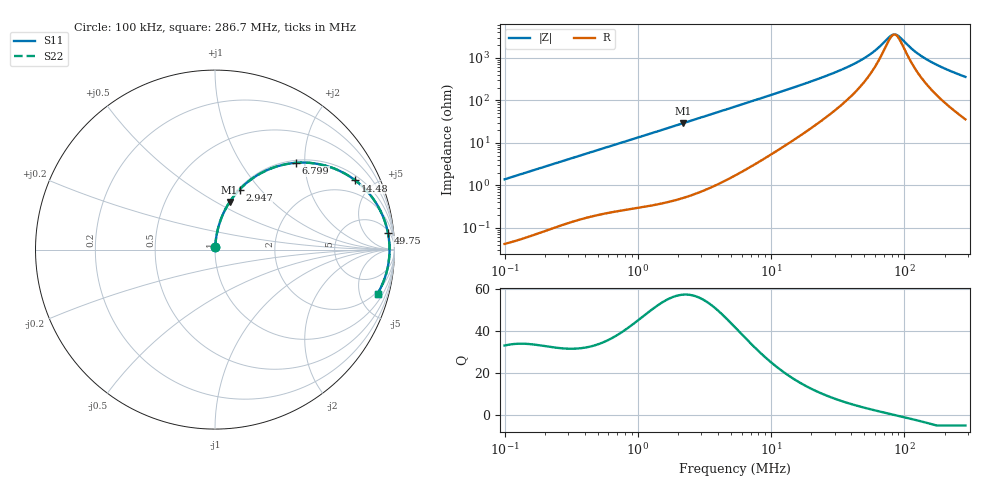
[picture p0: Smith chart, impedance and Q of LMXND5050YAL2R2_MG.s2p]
! LMXND5050YAL2R2_MG  S-PARAMETER MODEL  ( General Type )
! Model Generated by TAIYO YUDEN Corporation (http://www.ty-top.com)
! Version 1.0
! TAIYO YUDEN Control No. 191023NI43SB-FBB
! Copyright(c) 2019 TAIYO YUDEN CO.,LTD. All Rights Reserved.
! Product Description (link to TY-COMPAS)
! https://ds.yuden.co.jp/TYCOMPAS/or/detail?pn=LMXND5050YAL2R2NMG&u=M
! Products Name : Inductors
! Characteristics :
!  Inductance : 2.2 uH , SRF(min) : 42 MHz , DC Resistance(max) : 0.0286 Ohm
!  Rated Current : Saturation :5000 mA , Temp Rise : 3700 mA
!  Case Size : 4.9 x 4.9 / 0.193 x 0.193 [mm/inch] , Thickness : 4.1 / 0.161 [mm/inch]
!  (Conditions: Temperature = 25 degC , DC Bias Current/Voltage = 0A / 0V)
! External Node Assignments :
!  1  o---GGG---o  2
! GND o---------o GND
! Frequency Range : 0.1MHz  -  286.687601MHz  [ 402 STEP ]
# MHz S RI R 50
! Freq[MHz].  S11 Real  S11 Imag  S21 Real  S21 Imag  S12 Real  S12 Imag  S22 Real  S22 Imag
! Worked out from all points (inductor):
!   401 points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, 100 kHz to 286.7 MHz, reference 50 ohm
!   read as one part in series: L = 2.2 uH near 104.1 kHz
!   highest Q = 57.4 at 2.186 MHz (marker M1), where L = 2.11 uH
!   self-resonance near 84.18 MHz
!   S11 on the Smith chart (normalised r, x): 100 kHz: 1.00, +0.03; 2.947 MHz: 1.01, +0.78; 6.799 MHz: 1.05, +1.81; 14.48 MHz: 1.22, +3.93; 49.75 MHz: 6, +19; 286.7 MHz: 1.71, -7.08
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0.1  0.00061 0.0138  0.9994 -0.0138  0.9994 -0.0138  0.00061 0.0138
0.379416  0.00423 0.0511  0.9958 -0.0511  0.9958 -0.0511  0.00423 0.0511
0.776753  0.0131 0.102  0.9869 -0.102  0.9869 -0.102  0.0131 0.102
1.439567  0.0384 0.1829  0.9616 -0.1829  0.9616 -0.1829  0.0384 0.1829
2.186482  0.0812 0.2646  0.9188 -0.2646  0.9188 -0.2646  0.0812 0.2646
2.947127  0.1365 0.3345  0.8635 -0.3345  0.8635 -0.3345  0.1365 0.3345
3.972388  0.2215 0.4053  0.7785 -0.4053  0.7785 -0.4053  0.2215 0.4053
5.354322  0.339 0.4616  0.661 -0.4616  0.661 -0.4616  0.339 0.4616
6.798713  0.4511 0.4835  0.5489 -0.4835  0.5489 -0.4835  0.4511 0.4835
9.536008  0.6151 0.4679  0.3849 -0.4679  0.3849 -0.4679  0.6151 0.4679
14.48373  0.782 0.3853  0.218 -0.3853  0.218 -0.3853  0.782 0.3853
20.31517  0.8709 0.297  0.1291 -0.297  0.1291 -0.297  0.8709 0.297
34.08411  0.9418 0.17  0.0582 -0.17  0.0582 -0.17  0.9418 0.17
49.74838  0.9636 0.0928  0.0364 -0.0928  0.0364 -0.0928  0.9636 0.0928
60.70356  0.9693 0.0564  0.0307 -0.0564  0.0307 -0.0564  0.9693 0.0564
77.07906  0.9723 0.015  0.0277 -0.015  0.0277 -0.015  0.9723 0.015
83.46618  0.9726 0.00143  0.0274 -0.00143  0.0274 -0.00143  0.9726 0.00143
88.6015  0.9725 -0.00873  0.0275 0.00873  0.0275 0.00873  0.9725 -0.00873
117.0713  0.9692 -0.0569  0.0308 0.0569  0.0308 0.0569  0.9692 -0.0569
145.7234  0.9628 -0.0971  0.0372 0.0971  0.0372 0.0971  0.9628 -0.0971
200.3667  0.9448 -0.162  0.0552 0.162  0.0552 0.162  0.9448 -0.162
286.6876  0.9055 -0.2464  0.0945 0.2464  0.0945 0.2464  0.9055 -0.2464
